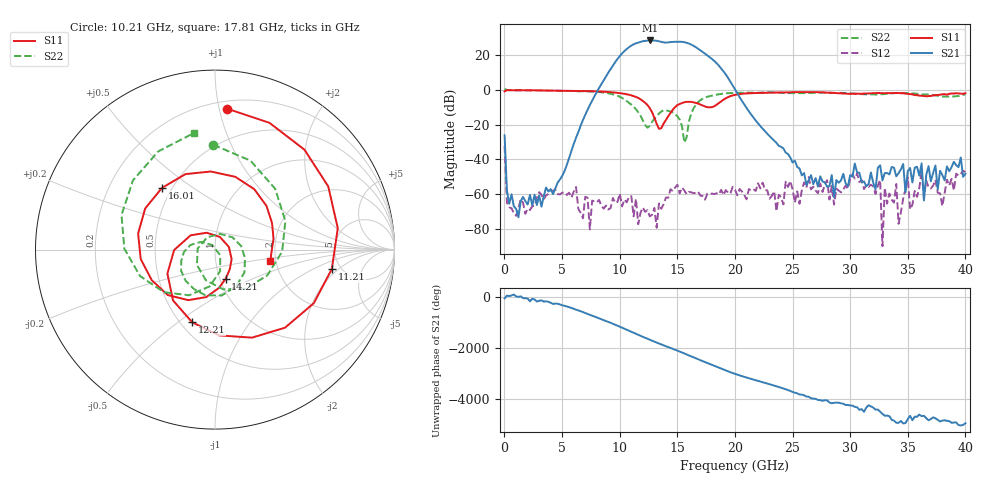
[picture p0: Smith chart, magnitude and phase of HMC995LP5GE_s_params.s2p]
!Agilent Technologies,E8361A,US43140893,A.06.04.32
!Agilent HMC995LP5GE: A.06.04.32
!Date: Wednesday, November 18, 2012 13:50:33
!Correction: S11(Full 2 Port(1,2)) S21(Full 2 Port(1,2)) S12(Full 2 Port(1,2)) S22(Full 2 Port(1,2))
!S2P File: Measurements: S11, S21, S12, S22:
# GHz S  dB  R 50
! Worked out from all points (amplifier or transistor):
!   201 points, 10 MHz to 40 GHz, reference 50 ohm
!   highest |S21| = 28.4 dB at 12.61 GHz (marker M1)
!   |S21| within 3 dB of that: 10.99 GHz to 16.38 GHz (5.382 GHz wide, 39.3 % of centre)
!   unconditionally stable (mu >= 1): 173.7 MHz to end of sweep
!   at 6.608 GHz: K = 439.47, MAG = -4.4 dB, |S12| = -70.7 dB
!   at 20 GHz: K = 59.22, MAG = 8.1 dB, |S12| = -57.4 dB
!   at 40 GHz: K = 4826.96, MAG = -40.3 dB, |S12| = -47.3 dB
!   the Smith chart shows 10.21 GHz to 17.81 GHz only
!   S11 on the Smith chart (normalised r, x): 10.21 GHz: 0.26, +1.06; 11.21 GHz: 4.23, -1.62; 12.21 GHz: 0.57, -0.57; 14.21 GHz: 1.07, -0.36; 16.01 GHz: 0.44, +0.38; 17.81 GHz: 1.87, -0.25
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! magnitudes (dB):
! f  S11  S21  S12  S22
! 10 MHz  -0.9  -26.2  -32.2  0.6
! 209.9 MHz  -0.2  -57.8  -65.0  -0.1
! 1.21 GHz  -0.2  -73.3  -68.3  -0.2
! 6.808 GHz  -0.7  -17.4  -73.9  -0.8
! 10.21 GHz  -2.1  21.0  -67.0  -4.7
! 11.21 GHz  -3.6  26.2  -72.8  -9.8
! 12.21 GHz  -7.4  28.1  -70.2  -20.3
! 12.61 GHz  -10.5  28.4  -72.8  -20.7
! 13.41 GHz  -22.4  27.9  -65.4  -13.6
! 14.21 GHz  -15.2  27.3  -62.1  -12.1
! 16.01 GHz  -6.9  26.6  -58.7  -18.1
! 17.81 GHz  -10.0  18.8  -60.0  -3.6
! 20.2 GHz  -2.7  -2.0  -60.7  -1.8
! 26.8 GHz  -1.3  -54.2  -55.7  -1.7
! 32.6 GHz  -1.9  -43.4  -51.9  -2.6
! 32.8 GHz  -1.9  -52.1  -89.9  -2.5
! 33.4 GHz  -1.9  -48.7  -59.7  -2.1
! 34 GHz  -1.8  -49.8  -54.2  -1.9
! 34.2 GHz  -1.8  -48.0  -77.1  -1.8
! 35 GHz  -2.2  -46.7  -50.5  -1.9
! 35.2 GHz  -2.5  -44.9  -68.7  -2.0
! 40 GHz  -1.9  -48.3  -47.3  -2.6
